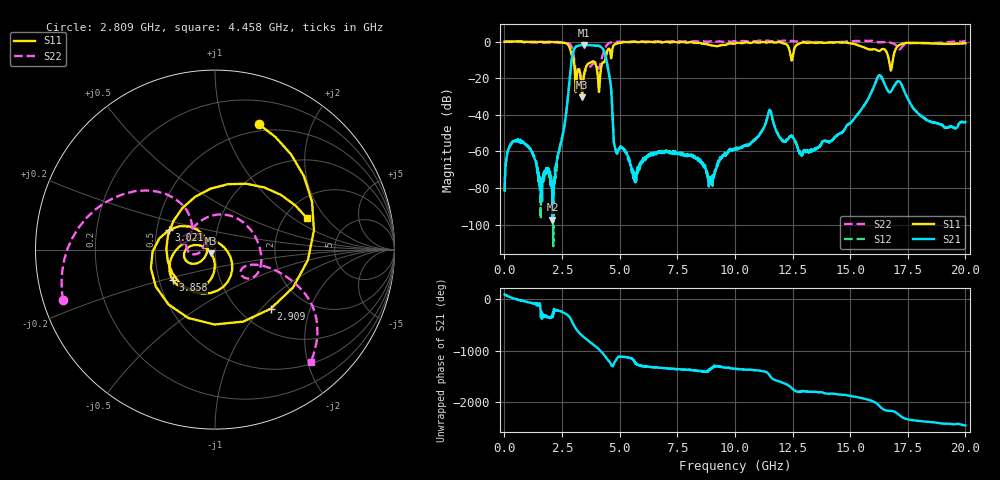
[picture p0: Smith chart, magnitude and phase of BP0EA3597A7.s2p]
! 9/17/2020 12:52:16 PM
! C:\ANRITSUVNA\DATA\MLO\SAMPLES\RAYTHEOM BP\17372_20GH_91720 .S2P
! CHANNEL.1
! TR.MEASUREMENT
! CORRECTED.DATA
# GHZ S RI R 50.0
! FREQ.GHZ  S11RE  S11IM  S31RE  S31IM  S13RE  S13IM  S33RE  S33IM
!; PortSelection: Port_13
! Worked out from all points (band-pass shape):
!   1601 points, 10 MHz to 20 GHz, reference 50 ohm
!   highest |S21| = -1.78 dB at 3.458 GHz (marker M1); lowest = -97.3 dB at 2.084 GHz (marker M2)
!   |S21| within 3 dB of the highest: 3.008 GHz to 4.308 GHz (1.3 GHz wide, 35.5 % of centre)
!   lowest |S11| = -30.4 dB at 3.371 GHz (marker M3), VSWR 1.06, Z = 47.7 - j1.88 ohm
!   |S11| at or under -10 dB: 3.009 GHz to 4.371 GHz (1.363 GHz wide, 36.9 % of centre); 12.4526 GHz to 12.4826 GHz (30 MHz wide, 0.241 % of centre); 16.68 GHz to 16.85 GHz (166.9 MHz wide, 0.996 % of centre)
!   |S22| runs from -23.8 to 0.6 dB; largest |S21 - S12| = 0.002
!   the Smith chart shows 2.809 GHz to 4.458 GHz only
!   S11 on the Smith chart (normalised r, x): 2.809 GHz: 0.43, +1.32; 2.909 GHz: 1.36, -1.13; 3.021 GHz: 0.58, +0.14; 3.858 GHz: 0.59, -0.22; 4.458 GHz: 2.63, +1.31
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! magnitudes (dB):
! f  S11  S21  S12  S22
! 10 MHz  0.0  -80.7  -82.1  0.0
! 597.2 MHz  0.1  -53.8  -53.8  -0.2
! 2.084 GHz  -0.3  -97.3  -89.2  -0.6
! 2.809 GHz  -2.6  -23.6  -23.5  -1.0
! 2.909 GHz  -6.9  -11.1  -11.1  -2.6
! 3.021 GHz  -11.1  -4.3  -4.3  -8.8
! 3.346 GHz  -26.1  -1.9  -1.9  -22.3
! 3.371 GHz  -30.4  -1.8  -1.8  -23.8
! 3.458 GHz  -17.7  -1.8  -1.8  -18.1
! 3.858 GHz  -10.8  -2.1  -2.1  -11.8
! 4.108 GHz  -27.5  -2.3  -2.3  -14.7
! 4.458 GHz  -5.3  -12.1  -12.1  -1.7
! 4.858 GHz  -1.1  -60.6  -60.7  -0.1
! 5.645 GHz  -0.1  -74.6  -74.4  -0.1
! 6.682 GHz  -0.1  -60.4  -60.9  0.0
! 8.943 GHz  -2.0  -77.1  -76.3  0.2
! 10.01 GHz  -1.0  -58.9  -58.1  0.2
! 11.52 GHz  -0.2  -37.3  -37.2  0.3
! 13.34 GHz  -0.4  -59.7  -59.0  -0.3
! 16.24 GHz  -5.1  -18.5  -18.5  -0.4
! 16.68 GHz  -9.7  -27.4  -27.4  -0.3
! 20 GHz  -0.9  -44.0  -43.9  0.2
